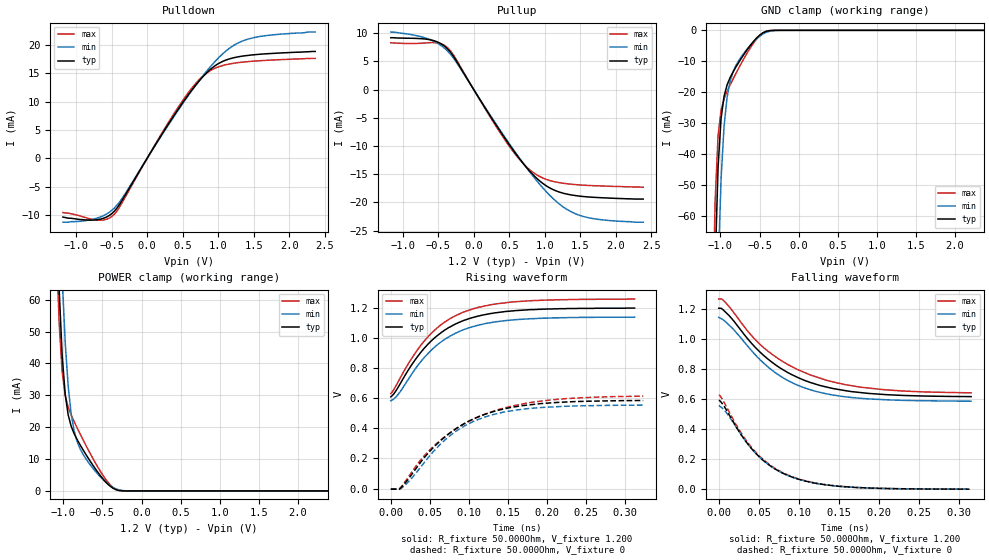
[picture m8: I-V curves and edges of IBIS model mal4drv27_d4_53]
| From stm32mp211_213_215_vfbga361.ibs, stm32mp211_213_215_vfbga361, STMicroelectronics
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[Model] mal4drv27_d4_53
Model_type   I/O
Polarity   Non-Inverting
Enable   Active-High
C_comp   1.656pF   1.652pF   1.661pF
C_comp_pullup   829.373fF   822.555fF   836.725fF
C_comp_pulldown 737.416fF   735.607fF   748.448fF
Vinh = 966.000mV
Vinl = 851.000mV
Vmeas = 909.000mV
Vref = 1.200V
Rref = 50Ohms
Cref = 0pF
[Model Spec]
Vinh   966.000mV   921.000mV   1.012V
Vinl   851.000mV   806.000mV   897.000mV
Vmeas   909.000mV   863.000mV   954.000mV
Vref   1.200V   1.140V   1.260V
D_overshoot_ampl_h 0.24 NA   NA
D_overshoot_ampl_l 0.24 NA   NA
D_overshoot_area_l 300.000m NA   NA
D_overshoot_area_h 300.000m NA   NA
[Receiver Thresholds]
Vth = 909.000mV
Vth_min = 863.000mV
Vth_max = 954.000mV
Vinh_ac = 68.000mV
Vinh_dc = 68.000mV
Vinl_ac = -68.000mV
Vinl_dc = -68.000mV
Tslew_ac = 5.000ns
Threshold_sensitivity = 0.5
Reference_supply Pullup_ref
[Temperature Range]   25.000   125.000   -40.000
[Voltage Range]   1.200V   1.140V   1.260V
[GND Clamp Reference]   0.00V   0.00V   0.00V
[C Comp Corner]
| variable   typ   min   max
C_comp 1.661pF   1.656pF   1.652pF
C_comp_pullup 829.373fF   836.725fF   822.555fF
C_comp_pulldown 735.607fF   748.448fF   737.416fF
[Pulldown Reference]   0.00V   0.00V   0.00V
[POWER Clamp Reference]   1.200V   1.140V   1.260V
[Pullup Reference]   1.200V   1.140V   1.260V
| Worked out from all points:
|   slope of the pulldown table from 0 to 0.18 V, typ, clamps not added: 49.1 ohm
|   slope of the pullup table from 0 to 0.18 V, typ, clamps not added: 49.4 ohm
|   GND clamp passes 1 mA (typ) near -0.47 V on its own axis
|   POWER clamp passes 1 mA (typ) near -0.37 V on its own axis
|   rising waveform, R_fixture 50.000Ohm, V_fixture 1.200: 20-80 % time 62.9ps typ, 62.7ps min, 63.2ps max; typ from 0.61 V to 1.2 V
|   rising waveform, R_fixture 50.000Ohm, V_fixture 0: 20-80 % time 78.2ps typ, 71.5ps min, 90.5ps max; typ from -0.004 V to 0.585 V
|   falling waveform, R_fixture 50.000Ohm, V_fixture 1.200: 20-80 % time 79.1ps typ, 72.5ps min, 87.7ps max; typ from 1.2 V to 0.615 V
|   falling waveform, R_fixture 50.000Ohm, V_fixture 0: 20-80 % time 60.2ps typ, 60.2ps min, 60.3ps max; typ from 0.589 V to 0 V
[GND Clamp]
-1.184V   -313.6mA   -372.3mA   -285.9mA
-1.107V   -133mA     -190.9mA   -103.4mA
-1.069V   -76.66mA   -125mA     -55.43mA
-1.031V   -44.19mA   -77.99mA   -34.02mA
-992.7mV  -28.51mA   -48.19mA   -25.88mA
-954.6mV  -21.35mA   -31.1mA    -22.21mA
-916.4mV  -17.7mA    -21.78mA   -19.79mA
-878.2mV  -15.35mA   -16.61mA   -17.73mA
-801.8mV  -11.82mA   -11.34mA   -13.9mA
-610.9mV  -4.628mA   -4.618mA   -5.371mA
-458.2mV  -822.8uA   -1.198mA   -809uA
2.367V    18.95nA    454.6nA    6.243nA
[Power Clamp]
-1.167V   171.5mA    206.4mA    156.1mA
-1.091V   92.44mA    126.6mA    77.99mA
-1.053V   63.02mA    93.75mA    52.4mA
-1.015V   42.49mA    66.9mA     37.37mA
-976.4mV  30.34mA    46.72mA    30.02mA
-938.2mV  23.88mA    32.9mA     26.3mA
-900mV    20.31mA    24.15mA    23.84mA
-823.6mV  16.11mA    15.49mA    19.79mA
-747.3mV  12.87mA    11.46mA    16.02mA
-518.2mV  4.545mA    4.187mA    5.836mA
-365.4mV  856.5uA    1.078mA    1.107mA
2.384V    -12.74nA   -415.5nA   -4.625nA
[Pulldown]
-1.184V   -10.3mA    -11.2mA    -9.5mA
-725.5mV  -10.8mA    -10.57mA   -10.79mA
-572.7mV  -10.31mA   -9.789mA   -10.69mA
-458.2mV  -9.247mA   -8.692mA   -9.771mA
-343.6mV  -7.212mA   -6.886mA   -7.612mA
458.2mV   9.017mA    8.853mA    9.379mA
687.3mV   12.92mA    12.9mA     13.22mA
878.2mV   15.51mA    15.93mA    15.34mA
1.145V    17.44mA    19.23mA    16.56mA
1.375V    18.04mA    20.78mA    16.96mA
1.756V    18.45mA    21.7mA     17.29mA
2.367V    18.8mA     22.2mA     17.58mA
[Pullup]
-1.167V   9.2mA      10.2mA     8.3mA
-670.9mV  8.955mA    9.121mA    8.283mA
-480mV    8.267mA    7.996mA    8.186mA
-365.4mV  7.194mA    6.806mA    7.397mA
-289.1mV  5.961mA    5.657mA    6.215mA
207.3mV   -4.186mA   -4.069mA   -4.35mA
550.9mV   -10.66mA   -10.5mA    -10.9mA
780mV     -14.35mA   -14.46mA   -14.13mA
1.047V    -17.27mA   -18.46mA   -16.02mA
1.276V    -18.42mA   -20.95mA   -16.63mA
1.505V    -18.91mA   -22.35mA   -16.91mA
2.384V    -19.4mA    -23.5mA    -17.3mA
[Ramp]
R_load=50.000Ohm
dV/dt_r   352.050mV/72.000ps  333.449mV/68.500ps  372.270mV/78.500ps
dV/dt_f   352.050mV/71.000ps  333.449mV/68.000ps  372.270mV/75.500ps
[Rising waveform]
R_fixture=50.000Ohm
V_fixture=1.200
V_fixture_min=1.140
V_fixture_max=1.260
0s        609.6mV    583.6mV    631.3mV
5ps       637.7mV    600.9mV    668.3mV
11ps      687.9mV    636.5mV    726.6mV
26ps      817.5mV    755.5mV    859.9mV
44ps      940.1mV    878mV      988.2mV
66ps      1.043V     981.3mV    1.096V
90ps      1.111V     1.05V      1.167V
119ps     1.155V     1.095V     1.213V
158ps     1.182V     1.122V     1.242V
312ps     1.2V       1.14V      1.26V
[Rising waveform]
R_fixture=50.000Ohm
V_fixture=0
0s        -4.294mV   -2.641mV   -2.653mV
11ps      -4.294mV   -2.641mV   -2.653mV
19ps      40.18mV    25.59mV    50.93mV
42ps      200.7mV    168.6mV    212.9mV
67ps      333.5mV    312.2mV    336.2mV
91ps      422.9mV    406.2mV    421.3mV
120ps     493.2mV    474.8mV    493.6mV
152ps     537.5mV    515.2mV    544.9mV
197ps     566.9mV    540.5mV    585.1mV
323ps     585.4mV    554.5mV    614.5mV
[Falling waveform]
R_fixture=50.000Ohm
V_fixture=1.200
V_fixture_min=1.140
V_fixture_max=1.260
0s        1.202V     1.141V     1.263V
4ps       1.198V     1.131V     1.263V
9ps       1.175V     1.11V      1.237V
39ps      980.6mV    932mV      1.031V
58ps      879.4mV    828.2mV    931.5mV
81ps      790.7mV    737.6mV    844.8mV
113ps     711.2mV    662.4mV    761.5mV
156ps     656.3mV    615.2mV    696.3mV
198ps     631.9mV    596.5mV    664.8mV
315ps     615.1mV    584.7mV    640mV
[Falling waveform]
R_fixture=50.000Ohm
V_fixture=0
0s        589.4mV    556.3mV    624mV
4ps       571.5mV    540.3mV    601.5mV
11ps      513.6mV    498.3mV    532.9mV
29ps      354mV      352.6mV    364.9mV
46ps      239.9mV    239mV      246.7mV
66ps      149.2mV    148.7mV    153.4mV
90ps      83.73mV    83.1mV     85.86mV
119ps     41.49mV    41.09mV    42.04mV
162ps     14.61mV    14.48mV    14.53mV
313ps     306.3uV    344.8uV    331.6uV
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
